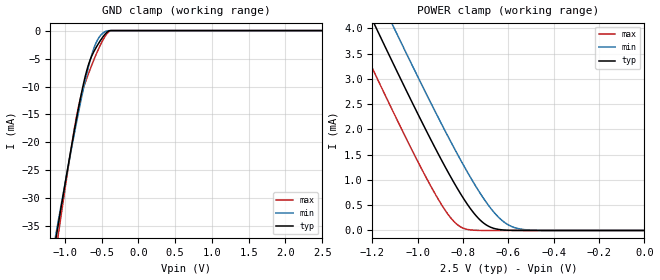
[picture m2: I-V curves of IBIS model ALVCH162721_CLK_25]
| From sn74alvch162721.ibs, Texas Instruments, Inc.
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[Model]   ALVCH162721_CLK_25
Model_type  Input
Vinl = 0.7
Vinh = 1.7
| variable   typ   min   max
C_comp   1.92pF   1.72pF   2.15pF
[Temperature Range]   40   100   -40
| Ambient temperature   25   85   -40
[Voltage range]   2.5   2.3   2.7
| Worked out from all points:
|   GND clamp passes 1 mA (typ) near -0.48 V on its own axis
|   POWER clamp passes 1 mA (typ) near -0.85 V on its own axis
[GND Clamp]
| ALVCH162721_CLK_25
|   Voltage   I(typ)   I(min)   I(max)
-2.5V     -153.1mA   -143.6mA   -168.5mA
-1.145V   -38.97mA   -38mA      -41.38mA
-1.11V    -36.17mA   -35.41mA   -38.21mA
-1.08V    -33.78mA   -33.21mA   -35.51mA
-895mV    -19.51mA   -19.99mA   -19.35mA
-800mV    -12.78mA   -13.61mA   -12.64mA
-700mV    -6.981mA   -7.539mA   -8.412mA
-615mV    -3.968mA   -3.483mA   -5.497mA
-540mV    -2.234mA   -1.292mA   -3.196mA
-450mV    -586.7uA   -156.6uA   -959.9uA
-375mV    -85.17nA   -8.524uA   -4.38uA
2.5V      34.28pA    152.6pA    32.5pA
[POWER Clamp]
| ALVCH162721_CLK_25
|   Voltage   I(typ)   I(min)   I(max)
-2.5V     16.88mA    17.58mA    15.98mA
-1.3V     5.111mA    5.849mA    4.158mA
-1.255V   4.681mA    5.42mA     3.727mA
-1.18V    3.971mA    4.711mA    3.015mA
-1.11V    3.316mA    4.055mA    2.36mA
-940mV    1.776mA    2.501mA    856.4uA
-845mV    982.9uA    1.676mA    200.1uA
-795mV    611.2uA    1.266mA    38.41uA
-725mV    207uA      738.7uA    1.527uA
-625mV    11.21uA    186.8uA    11.91nA
-510mV    181.6nA    9.688uA    51.12pA
-31.15fV  4.712pA    6.41pA     4.886pA
